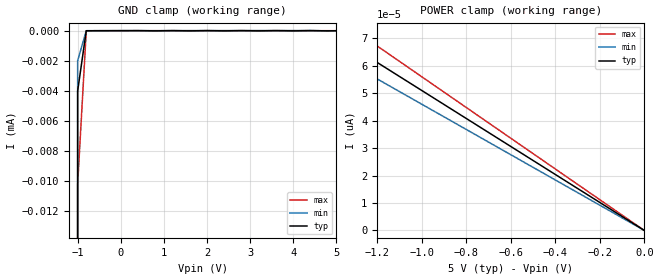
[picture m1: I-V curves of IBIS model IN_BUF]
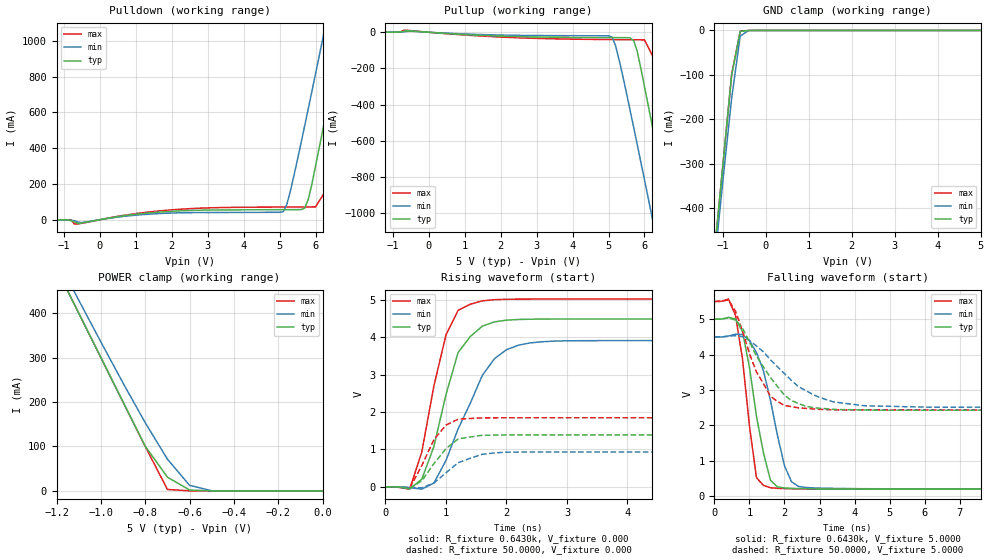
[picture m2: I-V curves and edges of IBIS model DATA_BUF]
| IBIS file m48z12.ibs created by s2ibis2 version 1.1
| North Carolina State University Electronics Research Laboratory  1995
[IBIS ver]   2.1
[File name]   m48z12.ibs
[File Rev]   0
[Date]   May 20, 2002
[Source]   ST models
[Copyright]   ST Microelectronics Inc.
|   Component m48z12 [Package]
[Component]   m48z12 [Package]
[Manufacturer]   ST Microelectronics
[Package]
| variable   typ   min   max
R_pkg   10.0000m   10.0000m   10.0000m
L_pkg   13.0000nH   8.0000nH   18.0000nH
C_pkg   6.0000pF   4.0000pF   8.0000pF
[Pin]  signal_name   model_name   R_pin   L_pin   C_pin
| fdatadummy   dummy
| goe  dummy   dummy
1   A7   IN_BUF
2   A6   IN_BUF
3   A5   IN_BUF
4   A4   IN_BUF
5   A3   IN_BUF
6   A2   IN_BUF
7   A1   IN_BUF
8   A0   IN_BUF
9   DQ0   DATA_BUF
10   DQ1   DATA_BUF
11   DQ2   DATA_BUF
12   VSS   GND
13   DQ3   DATA_BUF
14   DQ4   DATA_BUF
15   DQ5   DATA_BUF
16   DQ6   DATA_BUF
17   DQ7   DATA_BUF
18   E#   IN_BUF
19   A10   IN_BUF
20   G#   IN_BUF
21   W#   IN_BUF
22   A9   IN_BUF
23   A8   IN_BUF
24   VCC   POWER
[Package Model]  PCDIP24
| Models and submodels in the file (2): IN_BUF (Input), DATA_BUF (3-state)
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|   Model IN_BUF
[Model]   IN_BUF
Model_type   Input
Vinl =   0.8000V
Vinh =   2.0000V
C_comp   6.0800pF   5.9900pF   6.2200pF
[Temperature Range]   27.0000   0.000   70.0000
[Voltage Range]   5.0000V   4.5000V   5.5000V
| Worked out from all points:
|   GND clamp passes 1 mA (typ) near -1.03 V on its own axis
[GND_clamp]
| voltage   I(typ)   I(min)   I(max)
-5V       -3.645A    -3.66A     -3.622A
-1.2V     -6.986mA   -7.174mA   -6.983mA
-1V       -4.01uA    -1.994uA   -10.21uA
-800mV    -1.738nA   -399.5pA   -11.69nA
5V        5pA        5pA        372.3pA
[POWER_clamp]
| voltage   I(typ)   I(min)   I(max)
-5V       255pA      230pA      280pA
-1.6V     81.6pA     73.6pA     89.6pA
-1.5V     76.5pA     69pA       84pA
-1.4V     71.4pA     64.4pA     78.4pA
-1.3V     66.3pA     59.8pA     72.8pA
0V        0A         0A         0A
|   Model DATA_BUF
[Model]   DATA_BUF
Model_type   3-state
Polarity   Inverting
Enable   Active-Low
Vinl =   0.8000V
Vinh =   2.0000V
Vmeas =   1.5000V
Cref =1.000e-10F
Rref =   0.6430k
Vref =   1.7800V
C_comp   5.7000pF   5.6800pF   5.7700pF
[Temperature Range]   27.0000   0.000   70.0000
[Voltage Range]   5.0000V   4.5000V   5.5000V
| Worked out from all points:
|   slope of the pulldown table from 0 to 0.75 V, typ, clamps not added: 30.9 ohm
|   slope of the pullup table from 0 to 0.75 V, typ, clamps not added: 76.4 ohm
|   GND clamp passes 1 mA (typ) near -0.50 V on its own axis
|   POWER clamp passes 1 mA (typ) near -0.55 V on its own axis
|   rising waveform, R_fixture 0.6430k, V_fixture 0.000: 20-80 % time 440ps typ, 649ps min, 385ps max; typ from 0 V to 4.49 V
|   rising waveform, R_fixture 50.0000, V_fixture 0.000: 20-80 % time 417ps typ, 509ps min, 376ps max; typ from 0 V to 1.39 V
|   falling waveform, R_fixture 0.6430k, V_fixture 5.0000: 20-80 % time 495ps typ, 590ps min, 389ps max; typ from 5 V to 0.203 V
|   falling waveform, R_fixture 50.0000, V_fixture 5.0000: 20-80 % time 992ps typ, 1.37ns min, 750ps max; typ from 5 V to 2.43 V
[Pulldown]
| voltage   I(typ)   I(min)   I(max)
-5V       0A         0A         0A
-700mV    -12.42mA   -5.385mA   -24.43mA
1.9V      46.26mA    36.77mA    53.67mA
5.1V      56.32mA    44.77mA    71.05mA
5.3V      56.46mA    159.6mA    71.24mA
5.7V      65.01mA    526.4mA    71.6mA
6V        300mA      815.3mA    71.87mA
6.4V      700mA      1.206A     200mA
6.8V      1.1A       1.6A       600mA
7.2V      1.5A       2A         1A
7.6V      1.9A       2.4A       1.4A
10V       4.3A       4.8A       3.8A
[Pullup]
| voltage   I(typ)   I(min)   I(max)
-5V       0A         0A         0A
-700mV    4.708mA    1.83mA     11mA
5.1V      -29.62mA   -26.43mA   -40.57mA
5.3V      -29.79mA   -156.2mA   -40.9mA
5.7V      -46.98mA   -525.4mA   -41.47mA
5.8V      -107.4mA   -621.3mA   -41.6mA
6V        -300mA     -814.7mA   -42.12mA
6.4V      -700mA     -1.205A    -200mA
6.8V      -1.1A      -1.6A      -600mA
7.2V      -1.5A      -2A        -1A
7.6V      -1.9A      -2.4A      -1.4A
10V       -4.3A      -4.8A      -3.8A
[GND_clamp]
| voltage   I(typ)   I(min)   I(max)
-5V       -4.3A      -4.3A      -4.3A
-1.2V     -500mA     -524.6mA   -500mA
-1V       -300mA     -335.1mA   -300mA
-800mV    -100.6mA   -153.4mA   -100mA
-600mV    -2.081mA   -12.47mA   -1.528mA
-400mV    -2.338uA   -4.341uA   -113.9uA
5V        8.474nA    299.1uA    24.33nA
[POWER_clamp]
| voltage   I(typ)   I(min)   I(max)
-5V       4.3A       4.3A       4.3A
-1.2V     500mA      524.5mA    500mA
-1.1V     400mA      429.3mA    400mA
-900mV    200mA      242.6mA    200mA
-800mV    100.5mA    153.4mA    100mA
-700mV    30.92mA    71.4mA     3.297mA
-600mV    1.989mA    12.47mA    173.9uA
-500mV    44.72uA    299.1uA    14.9uA
0V        0A         0A         18.94nA
[Ramp]
| variable   typ   min   max
dV/dt_r   2.6914/0.4335n   2.3450/0.5812n   3.0112/0.3615n
dV/dt_f   2.8782/0.4273n   2.5731/0.5724n   3.1770/0.3578n
R_load = 0.6430k
[Rising Waveform]
R_fixture = 0.6430k
V_fixture = 0.000
V_fixture_min = 0.000
V_fixture_max = 0.000
| time   V(typ)   V(min)   V(max)
0s        3.115nV    3.324nV    12.02nV
400ps     -59.56mV   -21.83mV   -62.99mV
600ps     202.7mV    -63.39mV   928.1mV
800ps     1.073V     99.23mV    2.694V
1ns       2.466V     704.4mV    4.059V
1.2ns     3.589V     1.545V     4.718V
1.4ns     4.014V     2.228V     4.879V
1.8ns     4.409V     3.423V     5.002V
2.4ns     4.48V      3.849V     5.018V
10ns      4.486V     3.908V     5.019V
[Rising Waveform]
R_fixture = 50.0000
V_fixture = 0.000
V_fixture_min = 0.000
V_fixture_max = 0.000
| time   V(typ)   V(min)   V(max)
0s        2.133nV    2.174nV    8.435nV
200ps     -2.666mV   6.67uV     -8.046mV
400ps     -44.13mV   -16.91mV   -37.13mV
600ps     159.7mV    -26.17mV   567.6mV
800ps     616.7mV    101.4mV    1.259V
1ns       1.02V      373.6mV    1.65V
1.2ns     1.28V      643.5mV    1.806V
1.6ns     1.377V     868.3mV    1.842V
2ns       1.387V     926.1mV    1.844V
10ns      1.387V     930mV      1.845V
[Falling Waveform]
R_fixture = 0.6430k
V_fixture = 5.0000
V_fixture_min = 4.5000
V_fixture_max = 5.5000
| time   V(typ)   V(min)   V(max)
0s        5V         4.5V       5.5V
400ps     5.052V     4.525V     5.569V
600ps     5.006V     4.579V     5.111V
800ps     4.653V     4.568V     3.889V
1.2ns     2.258V     4.061V     526.5mV
1.4ns     1.226V     3.542V     310mV
1.6ns     455.2mV    2.707V     242.2mV
2ns       236.7mV    863mV      219.3mV
2.4ns     219mV      279.3mV    211.4mV
10ns      203mV      211.5mV    205.1mV
[Falling Waveform]
R_fixture = 50.0000
V_fixture = 5.0000
V_fixture_min = 4.5000
V_fixture_max = 5.5000
| time   V(typ)   V(min)   V(max)
0s        5V         4.5V       5.5V
400ps     5.037V     4.518V     5.545V
600ps     4.975V     4.537V     5.229V
800ps     4.749V     4.505V     4.672V
1.2ns     3.958V     4.244V     3.51V
1.6ns     3.35V      3.855V     2.824V
2ns       2.856V     3.464V     2.566V
3ns       2.488V     2.793V     2.458V
4.2ns     2.439V     2.564V     2.442V
10ns      2.432V     2.52V      2.44V
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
